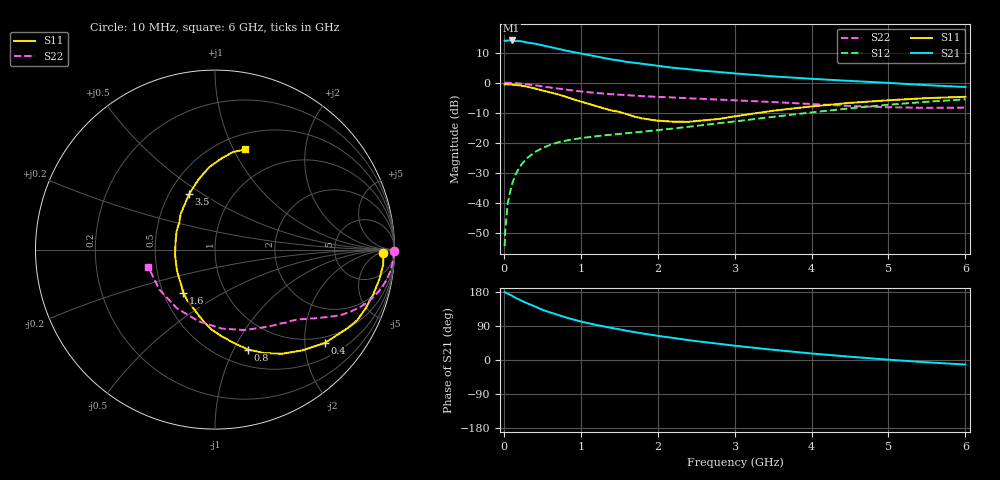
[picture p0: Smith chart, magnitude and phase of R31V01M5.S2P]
! SIEMENS Small Signal Semiconductors
! BFR181
! Si NPN RF Bipolar Junction Transistor in SOT23
! VCE = 1 V  IC = 1.5 mA
! Common Emitter S-Parameters:  May  1996
# GHz  S  MA  R  50
!  f  S11  S21  S12  S22
! GHz  MAG  ANG  MAG  ANG  MAG  ANG  MAG  ANG
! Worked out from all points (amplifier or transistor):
!   36 points, 10 MHz to 6 GHz, reference 50 ohm
!   highest |S21| = 14.1 dB at 100 MHz (marker M1)
!   |S21| within 3 dB of that: start of sweep to 743.3 MHz
!   unconditionally stable (mu >= 1): 1.668 GHz to 3.711 GHz
!   at 250 MHz: K = 0.20, MSG = 20.1 dB, |S12| = -26.6 dB
!   at 1.4 GHz: K = 0.91, MSG = 12.5 dB, |S12| = -17.3 dB
!   at 6 GHz: K = 0.90, MSG = 2.1 dB, |S12| = -5.5 dB
!   S11 on the Smith chart (normalised r, x): 10 MHz: 29, -9; 400 MHz: 0.84, -2.47; 800 MHz: 0.67, -1.14; 1.6 GHz: 0.63, -0.33; 3.5 GHz: 0.63, +0.44; 6 GHz: 0.66, +1.11
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0.01  0.9386 -1.1  5.037 179.3  0.0019 93.2  0.9973 -0.5
0.02  0.9395 -2.1  4.951 177.9  0.0037 87.6  0.9926 -1.0
0.05  0.9403 -5.3  5.043 175.1  0.0097 87.6  0.9962 -2.5
0.1  0.9301 -10.5  5.045 170.2  0.0195 83.2  0.9901 -5.1
0.15  0.9161 -15.7  4.923 164.3  0.0291 79.7  0.9815 -7.6
0.2  0.902 -21.0  4.928 159.5  0.0386 77.2  0.9708 -9.9
0.25  0.8847 -26.4  4.837 154.6  0.0468 73.8  0.9563 -12.4
0.4  0.8031 -40.4  4.467 141.6  0.0695 66.3  0.9078 -18.3
0.5  0.7419 -49.2  4.198 132.6  0.0815 61.6  0.8681 -21.7
0.6  0.6905 -57.2  3.929 125.7  0.0921 58.0  0.8321 -24.5
0.8  0.5864 -71.7  3.433 112.8  0.1083 52.4  0.7696 -28.7
0.9  0.5326 -78.3  3.242 106.9  0.1142 50.8  0.741 -30.3
1.1  0.4453 -92.6  2.901 97.1  0.1238 48.3  0.6933 -33.2
1.3  0.3734 -104.7  2.58 88.6  0.1327 47.1  0.6582 -35.6
1.6  0.2993 -126.4  2.216 77.0  0.1445 46.5  0.6202 -38.7
1.9  0.243 -150.2  1.989 67.1  0.1574 47.9  0.5883 -42.1
2.2  0.2244 -173.2  1.77 58.2  0.1725 48.6  0.5668 -45.9
2.8  0.2495 143.0  1.504 42.7  0.212 50.2  0.5233 -54.9
3.5  0.3413 115.1  1.274 27.0  0.2699 48.8  0.4764 -70.3
4.5  0.4614 93.9  1.069 8.7  0.3747 41.4  0.4095 -103.1
5.5  0.5534 79.5  0.909 -6.1  0.4811 29.1  0.3816 -144.3
6  0.5826 73.2  0.848 -11.9  0.5285 21.6  0.3842 -165.4
